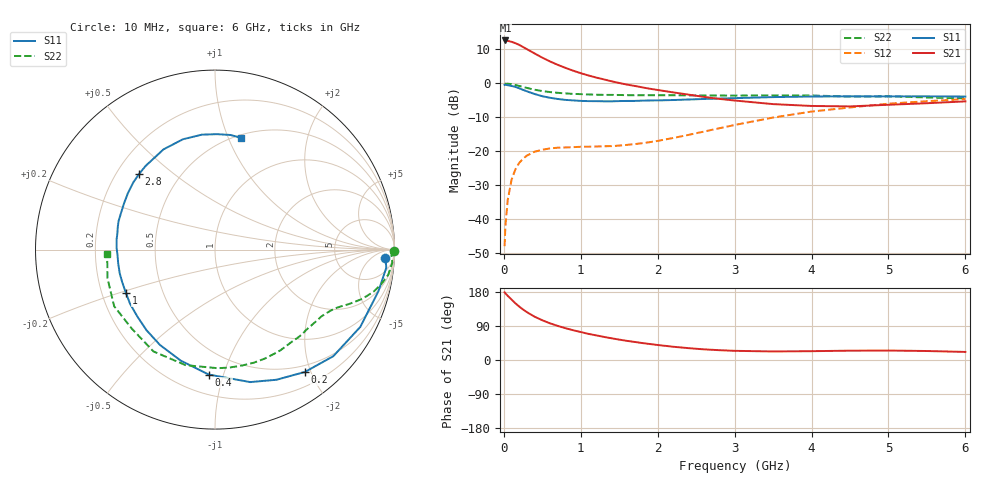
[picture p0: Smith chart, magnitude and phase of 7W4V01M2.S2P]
! Infineon Technologies  Discrete & RF Semiconductors
! BFS17W
! Si NPN RF Bipolar Junction Transistor in SOT323
! VCE = 4 V  IC = 1.2 mA
! Common Emitter S-Parameters:  August  1999
# GHz  S  MA  R  50
!  f  S11  S21  S12  S22
! GHz  MAG  ANG  MAG  ANG  MAG  ANG  MAG  ANG
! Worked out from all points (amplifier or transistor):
!   36 points, 10 MHz to 6 GHz, reference 50 ohm
!   highest |S21| = 12.6 dB at 20 MHz (marker M1)
!   |S21| within 3 dB of that: start of sweep to 334.2 MHz
!   unconditionally stable (mu >= 1): 989.5 MHz to end of sweep
!   at 250 MHz: K = 0.28, MSG = 16.5 dB, |S12| = -22.2 dB
!   at 1.4 GHz: K = 1.29, MAG = 6.3 dB, |S12| = -18.5 dB
!   at 6 GHz: K = 1.09, MAG = -2.2 dB, |S12| = -4.6 dB
!   S11 on the Smith chart (normalised r, x): 10 MHz: 20, -19; 200 MHz: 0.40, -1.91; 400 MHz: 0.33, -0.89; 1 GHz: 0.30, -0.21; 2.8 GHz: 0.29, +0.38; 6 GHz: 0.53, +1.11
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0.01  0.9497 -2.8  4.259 178.6  0.004 83.7  0.9999 -0.4
0.02  0.9599 -6.0  4.287 175.9  0.0078 87.6  0.9834 -1.6
0.05  0.9395 -14.3  4.232 169.4  0.019 82.6  0.9905 -4.3
0.1  0.917 -28.0  4.096 159.6  0.0379 73.9  0.9751 -8.3
0.15  0.8873 -42.0  3.907 149.7  0.0541 66.6  0.9456 -11.8
0.2  0.8459 -53.7  3.691 141.0  0.0674 60.5  0.9156 -14.7
0.25  0.802 -64.7  3.433 133.2  0.0777 54.8  0.8833 -17.1
0.3  0.7639 -75.1  3.19 126.3  0.0864 50.8  0.8563 -19.0
0.4  0.6969 -92.9  2.757 114.2  0.0985 43.8  0.806 -22.1
0.5  0.6469 -107.3  2.392 104.9  0.1052 39.1  0.7707 -24.2
0.6  0.6134 -120.0  2.105 96.8  0.1102 36.7  0.7447 -26.1
0.7  0.5894 -130.3  1.877 90.0  0.1128 34.8  0.7261 -28.1
0.8  0.5711 -139.3  1.694 84.0  0.1139 34.0  0.7119 -30.2
1  0.552 -154.0  1.412 73.8  0.1164 34.4  0.6941 -34.0
1.1  0.5478 -160.9  1.308 68.9  0.1166 35.2  0.6872 -36.5
1.6  0.5511 174.1  0.96 50.5  0.1241 44.4  0.6703 -48.7
2.2  0.5683 153.2  0.737 35.0  0.1569 58.4  0.6676 -65.4
2.8  0.597 135.2  0.591 25.9  0.218 64.6  0.662 -83.2
3.5  0.6278 117.2  0.495 22.5  0.3138 62.5  0.6643 -104.3
4.5  0.6446 96.5  0.458 24.6  0.4416 50.5  0.6393 -136.7
5.5  0.6444 82.3  0.51 23.7  0.5464 37.2  0.62 -165.2
6  0.6392 77.1  0.543 21.3  0.5861 31.0  0.6008 -177.7
